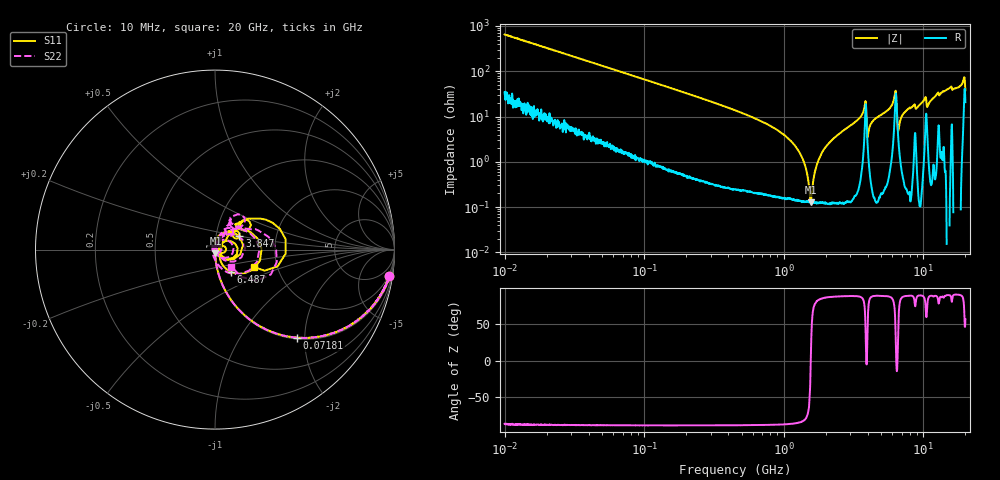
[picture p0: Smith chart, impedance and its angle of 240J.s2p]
!Keysight Technologies,P5008B,MY61100088,A.16.20.02
!Date: Tuesday, November 07, 2023 15:48:07
!Correction: S11(C  2-Port  )
!S21(C  2-Port  )
!S12(C  2-Port  )
!S22(C  2-Port  )
!S2P File: Measurements: S11, S21, S12, S22:Log Frequency Sweep
# Hz S  dB  R 50
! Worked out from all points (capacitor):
!   1601 points, 10 MHz to 20 GHz, reference 50 ohm
!   read as one part in series: C = 24.6 pF near 10.39 MHz
!   lowest |Z| = 128 mohm at 1.56 GHz (marker M1)
!   series resonance near 1.56 GHz, so ESL is about 420 pH
!   S11 on the Smith chart (normalised r, x): 10 MHz: 2, -13; 71.81 MHz: 1.03, -1.84; 3.847 GHz: 1.30, +0.20; 6.487 GHz: 1.16, -0.30; 20 GHz: 1.51, -0.31
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1e7  -0.17 -8.7  -16.38 78.3  -16.38 78.3  -0.17 -8.7
3.555162e7  -1.20 -28.3  -6.51 60.4  -6.51 60.4  -1.20 -28.3
7.181326e7  -3.46 -47.0  -2.73 42.0  -2.73 42.0  -3.46 -47.0
1.263918e8  -6.73 -61.9  -1.10 27.2  -1.11 27.2  -6.73 -61.9
4.472136e8  -16.98 -81.5  -0.11 7.5  -0.11 7.5  -16.98 -81.6
1.55999e9  -33.99 -82.7  -0.01 -1.1  -0.01 -1.1  -33.96 -91.9
1.589917e9  -34.55 -82.1  -0.01 -1.3  -0.01 -1.3  -34.53 -92.2
2.227705e9  -54.09 20.8  -0.01 -3.5  -0.01 -3.5  -58.26 -5.8
2.61821e9  -39.08 88.6  -0.01 -4.8  -0.01 -4.8  -39.56 64.4
3.846973e9  -16.20 28.4  -1.24 -11.5  -1.24 -11.5  -15.74 19.6
4.190402e9  -44.47 99.6  -0.03 -7.4  -0.03 -7.4  -38.81 20.2
4.521328e9  -33.21 94.6  -0.01 -9.1  -0.01 -9.1  -32.65 57.4
5.652411e9  -25.71 70.7  -0.04 -13.6  -0.04 -13.6  -25.28 68.7
6.487314e9  -16.26 -54.4  -0.82 -5.6  -0.82 -5.6  -17.09 -62.8
7.100103e9  -30.56 -30.2  -0.01 -13.0  -0.02 -13.0  -36.80 -161.3
8.5048e9  -28.93 30.3  -0.05 -18.9  -0.05 -18.8  -32.01 70.7
9.176444e9  -33.63 -0.1  0.01 -19.4  0.01 -19.3  -39.64 128.2
1.023592e10  -21.70 36.0  -0.22 -24.9  -0.22 -24.9  -22.94 50.0
1.109686e10  -29.41 19.3  -0.01 -23.2  -0.01 -23.2  -32.90 84.7
1.231939e10  -18.82 46.4  -0.06 -28.2  -0.06 -28.1  -19.12 67.4
1.387292e10  -14.39 44.5  -0.24 -31.7  -0.25 -31.6  -14.70 59.0
2e10  -12.49 -24.2  -1.88 -37.5  -1.88 -37.4  -17.55 -46.2
